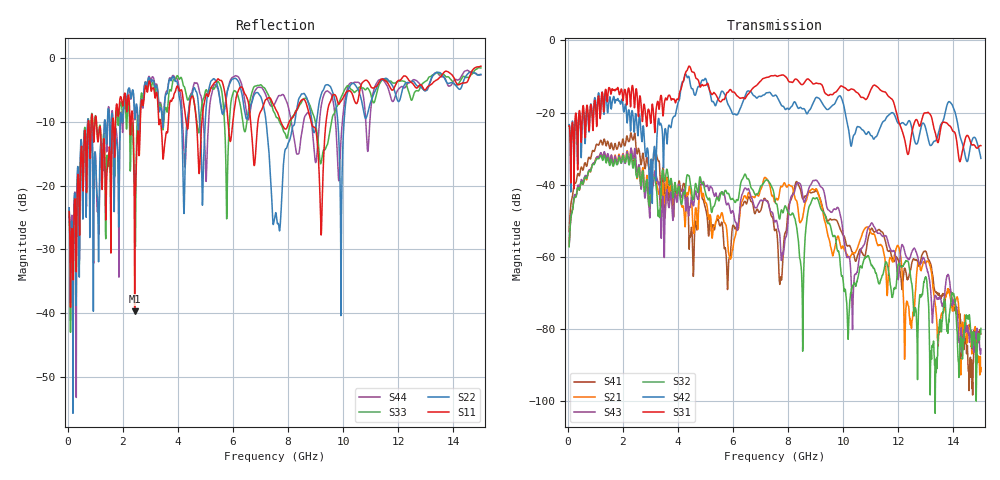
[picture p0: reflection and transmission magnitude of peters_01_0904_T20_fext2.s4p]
# MHZ S RI R 50.00
! FREQ  S11  S12  S13  S14
!  S21  S22  S23  S24
!  S31  S32  S33  S34
!  S41  S42  S43  S44
!  REAL  IMAG  REAL  IMAG  REAL  IMAG  REAL  IMAG
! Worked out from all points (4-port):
!   1496 points, 50 MHz to 15 GHz, reference 50 ohm
!   strongest paths, dB at 50 MHz, 3.79 GHz, 7.53 GHz, 11.27 GHz, 15 GHz:
!     S31: -23.7, -16.2, -9.7, -13.1, -29.2
!     S42: -23.3, -22.1, -15.2, -25.6, -32.7
!     S32: -57.3, -41.5, -44.7, -67.0, -79.9
!     S43: -56.9, -47.0, -50.3, -53.5, -85.7
!     S21: -57.0, -44.0, -44.7, -56.9, -90.9
!     S41: -53.0, -41.9, -52.7, -52.6, -81.4
!   lowest |S11| = -39.7 dB at 2.43 GHz (marker M1), VSWR 1.02, Z = 49 - j0.0201 ohm
!   |S11| at or under -10 dB: start of sweep to 743 MHz; 1.044 GHz to 1.625 GHz (581.5 MHz wide, 43.6 % of centre); 8.838 GHz to 9.379 GHz (540.8 MHz wide, 5.94 % of centre)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
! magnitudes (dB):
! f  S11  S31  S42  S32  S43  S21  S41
! 50 MHz  -24.1  -23.7  -23.3  -57.3  -56.9  -57.0  -53.0
! 2.43 GHz  -39.7  -18.5  -23.8  -32.7  -30.0  -31.0  -25.7
! 5.82 GHz  -10.0  -14.4  -17.7  -42.4  -45.1  -57.4  -66.0
! 7.18 GHz  -6.6  -10.3  -14.7  -38.8  -44.2  -38.1  -44.1
! 7.73 GHz  -9.9  -9.7  -17.6  -47.9  -57.8  -40.6  -65.6
! 8.32 GHz  -8.1  -10.8  -18.2  -52.2  -39.6  -44.7  -39.2
! 15 GHz  -1.3  -29.2  -32.7  -79.9  -85.7  -90.9  -81.4
